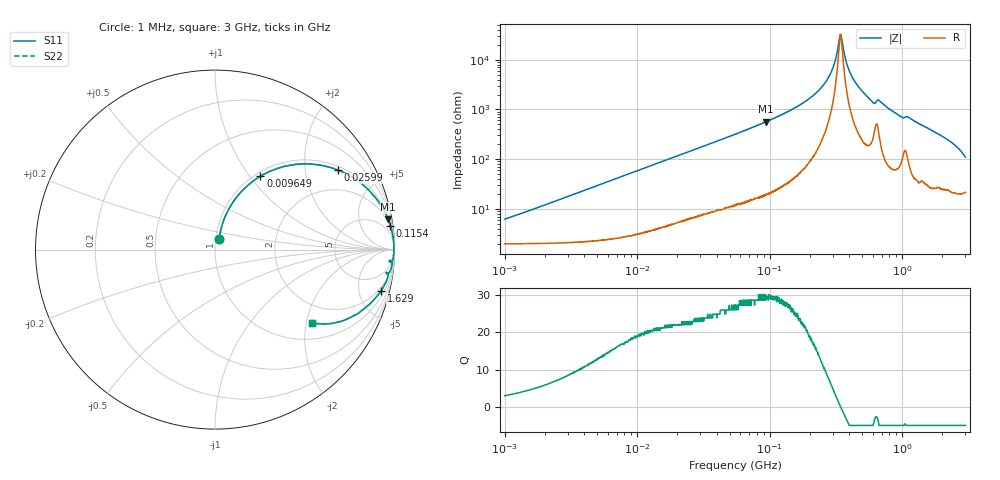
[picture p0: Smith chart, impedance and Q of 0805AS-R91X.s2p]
!s-Parameter Generated by FASTRON Sdn. Bhd.
!FASTRON P/N : 0805AS-R91X
!Keysight Technologies: E4991B_MY54100416_A.01.15
!Date: Mon Jun 15 12:56:21 2026
!Version  :Rev01  Mon Jun 15 12:56:21 2026
!Data & Calibration Information:
!Freq  S11  S21  S12  S22
!PortZ  Port1:50+j0  Port2:50+j0
!When reading reference impedance value at option line is always used.
! Remarks : This data is being provided solely for informational purposes.
# Hz S dB R 50
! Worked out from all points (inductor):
!   1601 points, 1 MHz to 3 GHz, reference 50 ohm
!   read as one part in series: L = 937 nH near 1.041 MHz
!   highest Q = 29.8 at 94.03 MHz (marker M1), where L = 964 nH
!   self-resonance near 341.9 MHz
!   S11 on the Smith chart (normalised r, x): 1 MHz: 1.04, +0.12; 9.649 MHz: 1.06, +1.13; 25.99 MHz: 1.13, +3.00; 115.4 MHz: 2, +14; 1.629 GHz: 1.53, -7.85; 3 GHz: 1.43, -2.15
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1000000  -24.30 68.2  -0.18 -3.3  -0.18 -3.3  -24.30 68.2
3804036  -13.40 72.1  -0.39 -12.3  -0.39 -12.3  -13.40 72.1
9648503  -6.36 58.3  -1.40 -28.7  -1.40 -28.7  -6.36 58.3
1.447069e7  -4.02 48.3  -2.53 -39.0  -2.53 -39.0  -4.02 48.3
2.598685e7  -1.77 32.9  -5.28 -54.5  -5.28 -54.5  -1.77 32.9
5.504702e7  -0.50 17.3  -10.50 -70.6  -10.50 -70.6  -0.50 17.3
9.402997e7  -0.18 9.9  -15.30 -78.1  -15.30 -78.1  -0.18 9.9
1.15443e8  -0.12 7.8  -17.30 -80.2  -17.30 -80.2  -0.12 7.8
2.083556e8  -0.04 3.1  -25.20 -83.6  -25.20 -83.6  -0.04 3.1
2.841474e8  -0.03 1.1  -33.90 -80.7  -33.90 -80.7  -0.03 1.1
3.062963e8  -0.03 0.7  -38.10 -75.1  -38.10 -75.1  -0.03 0.7
3.334925e8  -0.03 0.2  -47.40 -44.8  -47.40 -44.8  -0.03 0.2
3.436571e8  -0.03 -0.0  -50.20 4.1  -50.20 4.1  -0.03 -0.0
3.523638e8  -0.03 -0.2  -47.40 42.1  -47.40 42.1  -0.03 -0.2
3.91407e8  -0.03 -0.8  -36.80 76.0  -36.80 76.0  -0.03 -0.8
4.525341e8  -0.04 -1.8  -30.30 81.3  -30.30 81.3  -0.04 -1.8
5.959055e8  -0.12 -3.9  -23.20 76.4  -23.20 76.4  -0.12 -3.9
6.719458e8  -0.13 -3.7  -23.70 75.4  -23.70 75.4  -0.13 -3.7
7.925923e8  -0.10 -5.4  -20.50 80.7  -20.50 80.7  -0.10 -5.4
1.629261e9  -0.41 -14.0  -12.30 72.2  -12.30 72.2  -0.41 -14.0
2.371269e9  -1.17 -23.9  -7.81 60.4  -7.81 60.4  -1.17 -23.9
3e9  -3.41 -37.2  -4.21 41.5  -4.21 41.5  -3.41 -37.2
